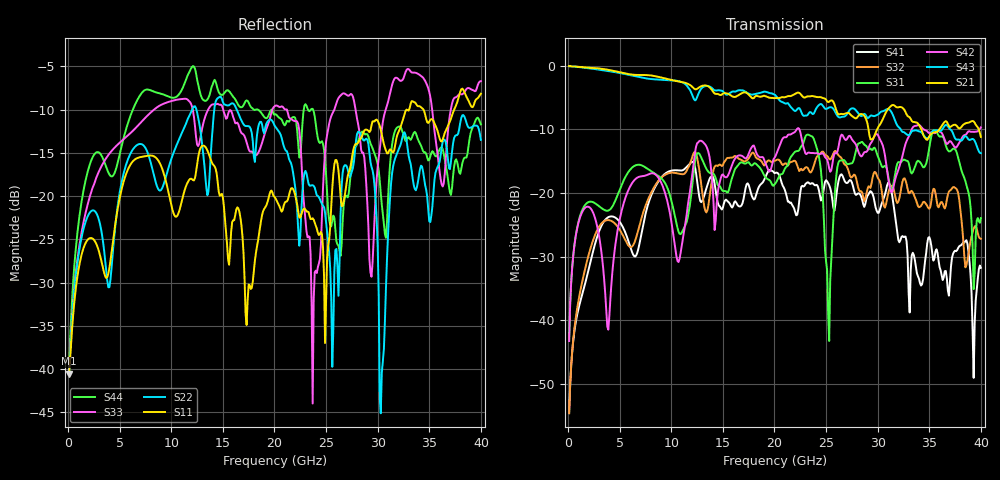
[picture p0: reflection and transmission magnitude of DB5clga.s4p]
! ADC12DJ3200QML-SP
! 196-pin ZMX package
! CLGA Ceramic Package without columns (ceramic land grid array)
! Texas Instruments 4/21/2021
! Single-ended  S-parameters
! PORT#  PORT_NAME  NET_NAME
! PORT1:  DAxN.DIEBUMP DAxN
! PORT2:  DAxN.BGA  DAxN
! PORT3:  DAxP.DIEBUMP DAxP
! PORT4:  DAxP.BGA  DAxP
! Touchstone Ver. 1.0
! Number of ports is 4
# Hz	S	MA	R	50.000000
! SCATTERING PARAMETERS  :
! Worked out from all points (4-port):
!   400 points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, 100 MHz to 40 GHz, reference 50 ohm
!   strongest paths, dB at 100 MHz, 10.1 GHz, 20.1 GHz, 30.1 GHz, 40 GHz:
!     S21: -0.1, -2.3, -5.1, -9.5, -11.2
!     S43: -0.1, -2.3, -4.7, -7.6, -13.7
!     S42: -43.3, -25.5, -14.2, -11.1, -9.7
!     S31: -43.2, -21.8, -18.5, -14.6, -23.9
!     S32: -54.6, -16.8, -14.9, -17.8, -27.2
!     S41: -54.6, -16.5, -16.8, -23.1, -31.8
!   lowest |S11| = -40.5 dB at 100 MHz (marker M1), VSWR 1.02, Z = 50.9 - j0.377 ohm
!   |S11| at or under -10 dB: start of sweep to 32.8 GHz; 32.8 GHz to 33.04 GHz (235.2 MHz wide, 0.715 % of centre); 34.43 GHz to 37.41 GHz (2.983 GHz wide, 8.31 % of centre)
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1e8  0.00941 -23.2  0.9908 -3.7  0.006903 77.6  0.001869 -129.6
     0.9908 -3.7  0.009636 -23.9  0.001861 -128.9  0.006877 76.4
     0.006903 77.6  0.001861 -128.9  0.009772 -30.6  0.9908 -3.8
     0.001869 -129.6  0.006877 76.4  0.9908 -3.8  0.01043 -30.2
4.9e9  0.09076 -60.9  0.8916 -175.0  0.1014 37.6  0.0607 54.2
       0.8916 -175.0  0.09611 -86.3  0.05303 45.4  0.0566 105.8
       0.1014 37.6  0.05303 45.4  0.2009 -41.0  0.8797 -176.7
       0.0607 54.2  0.0566 105.8  0.8797 -176.7  0.1645 -113.4
2.22e10  0.08912 81.3  0.6124 -35.2  0.2134 84.6  0.06738 179.3
         0.6124 -35.2  0.08255 123.3  0.165 138.7  0.3196 10.9
         0.2134 84.6  0.165 138.7  0.2697 -53.2  0.4548 -46.1
         0.06738 179.3  0.3196 10.9  0.4548 -46.1  0.2386 126.6
2.37e10  0.07443 -1.5  0.5767 -90.1  0.2755 21.9  0.1194 113.9
         0.5767 -90.1  0.1156 153.8  0.1541 104.4  0.2065 3.0
         0.2755 21.9  0.1541 104.4  0.006329 105.6  0.4168 -89.1
         0.1194 113.9  0.2065 3.0  0.4168 -89.1  0.3193 121.8
2.53e10  0.0561 -15.4  0.5213 -149.8  0.006885 162.3  0.1152 47.7
         0.5213 -149.8  0.04688 128.0  0.185 29.8  0.1559 0.8
         0.006885 162.3  0.185 29.8  0.2623 23.5  0.47 -146.7
         0.1152 47.7  0.1559 0.8  0.47 -146.7  0.07266 102.1
2.81e10  0.2034 -167.1  0.4006 122.3  0.2431 53.7  0.09927 -61.3
         0.4006 122.3  0.2354 -151.6  0.1112 -90.1  0.2143 -13.0
         0.2431 53.7  0.1112 -90.1  0.2618 -104.9  0.4246 116.2
         0.09927 -61.3  0.2143 -13.0  0.4246 116.2  0.2077 -174.1
4e10  0.3908 174.0  0.2756 60.8  0.0635 15.3  0.02583 -74.0
      0.2756 60.8  0.2113 -154.3  0.04368 -137.1  0.3276 -26.8
      0.0635 15.3  0.04368 -137.1  0.4619 -173.4  0.2054 79.4
      0.02583 -74.0  0.3276 -26.8  0.2054 79.4  0.2599 170.2
